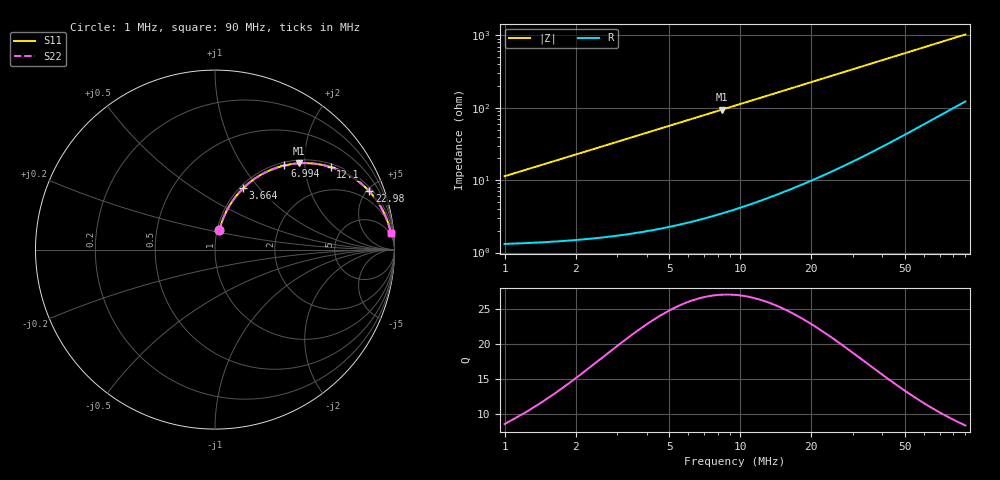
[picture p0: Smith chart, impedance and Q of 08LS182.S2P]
! Coilcraft 0805LS-182 Chip Inductor
! 18 September 2002
# MHZ S MA R 50
!Freq  MagS11  AngS11  MagS21  AngS21  MagS12  AngS12  MagS22  AngS22
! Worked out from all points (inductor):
!   402 points, 1 MHz to 90 MHz, reference 50 ohm
!   read as one part in series: L = 1.79 uH near 1.444 MHz
!   highest Q = 27.1 at 8.326 MHz (marker M1), where L = 1.79 uH
!   S11 on the Smith chart (normalised r, x): 1 MHz: 1.03, +0.22; 3.664 MHz: 1.04, +0.82; 6.994 MHz: 1.06, +1.57; 12.1 MHz: 1.10, +2.72; 22.98 MHz: 1.24, +5.19; 90 MHz: 3, +20
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1  0.1111 77.0  0.981 -6.3  0.981 -6.3  0.1111 77.0
1.222  0.135 76.7  0.9777 -7.7  0.9777 -7.7  0.135 76.7
1.888  0.2053 74.2  0.9647 -11.8  0.9647 -11.8  0.2053 74.2
2.332  0.2505 72.1  0.9534 -14.5  0.9534 -14.5  0.2505 72.1
2.998  0.3151 68.8  0.9333 -18.3  0.9333 -18.3  0.3151 68.8
3.664  0.3753 65.4  0.91 -22.0  0.91 -22.0  0.3753 65.4
4.33  0.431 62.1  0.8843 -25.5  0.8843 -25.5  0.431 62.1
5.218  0.4979 57.9  0.8477 -29.8  0.8477 -29.8  0.4979 57.9
6.994  0.6076 50.5  0.7719 -37.4  0.7719 -37.4  0.6076 50.5
8.326  0.6716 45.7  0.7166 -42.2  0.7166 -42.2  0.6716 45.7
10.102  0.7376 40.4  0.6485 -47.5  0.6485 -47.5  0.7376 40.4
12.1  0.7921 35.5  0.5812 -52.3  0.5812 -52.3  0.7921 35.5
13.876  0.828 31.9  0.5295 -55.8  0.5295 -55.8  0.828 31.9
15.874  0.8584 28.6  0.4797 -59.1  0.4797 -59.1  0.8584 28.6
19.204  0.8935 24.3  0.4123 -63.2  0.4123 -63.2  0.8935 24.3
22.978  0.919 20.7  0.354 -66.6  0.354 -66.6  0.919 20.7
30.748  0.9477 15.8  0.2722 -71.1  0.2722 -71.1  0.9477 15.8
37.852  0.961 12.9  0.2238 -73.6  0.2238 -73.6  0.961 12.9
45.622  0.9694 10.7  0.1869 -75.2  0.1869 -75.2  0.9694 10.7
60.496  0.9777 8.1  0.1418 -76.9  0.1418 -76.9  0.9777 8.1
75.37  0.9817 6.5  0.1142 -77.6  0.1142 -77.6  0.9817 6.5
90  0.9841 5.5  0.09586 -77.7  0.09586 -77.7  0.9841 5.5
